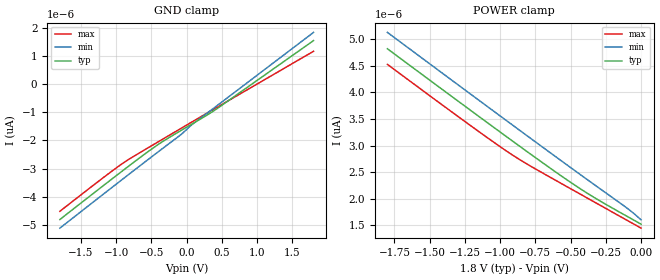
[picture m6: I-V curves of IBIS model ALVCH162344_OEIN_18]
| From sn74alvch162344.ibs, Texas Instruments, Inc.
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[Model]   ALVCH162344_OEIN_18
Model_type  Input
Vinl = 0.5775
Vinh = 1.2675
| variable   typ   min   max
C_comp   1.25pF   1.16pF   1.32pF
[Temperature Range]   40   100   -40
| Ambient temperature   25   85   -40
[Voltage range]   1.8   1.65   1.95
[GND Clamp]
| ALVCH162344_OEIN_18
|   Voltage   I(typ)   I(min)   I(max)
-1.8V     -4.821pA   -5.129pA   -4.527pA
-1.12V    -3.488pA   -3.792pA   -3.204pA
-825mV    -2.918pA   -3.216pA   -2.678pA
-360mV    -2.068pA   -2.319pA   -1.981pA
-85mV     -1.649pA   -1.795pA   -1.574pA
105mV     -1.367pA   -1.373pA   -1.293pA
425mV     -870.9fA   -766.1fA   -822.1fA
1.8V      1.567pA    1.859pA    1.186pA
[POWER Clamp]
| ALVCH162344_OEIN_18
|   Voltage   I(typ)   I(min)   I(max)
-1.8V     4.821pA    5.129pA    4.527pA
-1.195V   3.634pA    3.939pA    3.347pA
-890mV    3.043pA    3.343pA    2.785pA
-610mV    2.511pA    2.799pA    2.353pA
-415mV    2.161pA    2.424pA    2.063pA
-105mV    1.678pA    1.835pA    1.603pA
0V        1.523pA    1.603pA    1.448pA
